| IBIS file usssh2gxxac.ibs created by s2ibis3 verion 1.1
| North Carolina State University, ERL, 2006
| This Model is valid for Commercial Temperature Range 0C<=Tc<=95C
| Valid for DDR3-800/1066/1333/1600/1866 operation
| Part Number   VDD/VDDQ   Package   Architecture
| SCB15H2G160AF   1.5 +0.1/-0.1   96-Ball FBGA   128Meg x 16
| SCB15H2G800AF   1.5 +0.1/-0.1   78-Ball FBGA   256Meg x 8
| TOPR: Operating Temperature
[IBIS Ver]   3.2
[File name]  usssh2gxxac.ibs
[File Rev]   1.2
[Date]   2016-10-18
[Source]   Simulation of a silicon level SPICE model
[Notes]   IBIS Characteristics for I/O Buffer
   IBIS Model Revision History:
Rev 1.1: 2016-03-29
   - IBIS model file initial creation
Rev 1.2: 2016-10-18
   - updata company and other informations;
   - updata OCD rising falling data to support 1866MB frequency;
[disclaimer] The IBIS models are for modeling purpose only and are
   subject to change without any notice. UniIC is not
   responsible for any problems the models may cause.
[Copyright]  Copyright 2016 UniIC Corp. All rights reserved
|   Component SCB15H2G160AF
[Component]   SCB15H2G160AF
[Manufacturer]  UniIC Corp.
| All balls excluding NC, POWER and GND (R[Ohm], L[H], C[F])
[Package]   | 96-Ball FBGA
|Variable   typ   min   max
R_pkg   5.54E-01   4.56E-01   6.22E-01
L_pkg   1.97E-09   1.50E-09   2.61E-09
C_pkg   6.13E-13   3.99E-13   9.02E-13
[Pin] signal_name   model_name   R_pin   L_pin   C_pin
A1   VDDQ   POWER   NA   NA   NA
A2   DQU5   DQ   5.95E-01   1.95E-09   6.80E-13
A3   DQU7   DQ   5.58E-01   1.70E-09   7.16E-13
A7   DQU4   DQ   5.77E-01   1.84E-09   6.35E-13
A8   VDDQ   POWER   NA   NA   NA
A9   VSS   GND   NA   NA   NA
B1   VSSQ   GND   NA   NA   NA
B2   VDD   POWER   NA   NA   NA
B3   VSS   GND   NA   NA   NA
B7   DQSU#   DQ   5.85E-01   2.01E-09   6.55E-13
B8   DQU6   DQ   6.22E-01   2.08E-09   7.44E-13
B9   VSSQ   GND   NA   NA   NA
C1   VDDQ   POWER   NA   NA   NA
C2   DQU3   DQ   5.85E-01   2.21E-09   6.52E-13
C3   DQU1   DQ   5.65E-01   1.96E-09   6.71E-13
C7   DQSU   DQ   5.99E-01   2.17E-09   6.18E-13
C8   DQU2   DQ   5.52E-01   1.73E-09   6.58E-13
C9   VDDQ   POWER   NA   NA   NA
D1   VSSQ   GND   NA   NA   NA
D2   VDDQ   POWER   NA   NA   NA
D3   DMU   DM   5.80E-01   2.01E-09   5.99E-13
D7   DQU0   DQ   5.32E-01   1.62E-09   5.78E-13
D8   VSSQ   GND   NA   NA   NA
D9   VDD   POWER   NA   NA   NA
E1   VSS   GND   NA   NA   NA
E2   VSSQ   GND   NA   NA   NA
E3   DQL0   DQ   5.65E-01   1.98E-09   6.31E-13
E7   DML   DM   5.39E-01   1.73E-09   6.06E-13
E8   VSSQ   GND   NA   NA   NA
E9   VDDQ   POWER   NA   NA   NA
F1   VDDQ   POWER   NA   NA   NA
F2   DQL2   DQ   5.73E-01   2.13E-09   5.09E-13
F3   DQSL   DQ   5.04E-01   2.07E-09   5.92E-13
F7   DQL1   DQ   5.15E-01   1.65E-09   4.09E-13
F8   DQL3   DQ   5.71E-01   1.79E-09   6.63E-13
F9   VSSQ   GND   NA   NA   NA
G1   VSSQ   GND   NA   NA   NA
G2   DQL6   DQ   5.43E-01   1.97E-09   7.24E-13
G3   DQSL#   DQ   5.03E-01   1.93E-09   5.03E-13
G7   VDD   POWER   NA   NA   NA
G8   VSS   GND   NA   NA   NA
G9   VSSQ   GND   NA   NA   NA
H1   VREFDQ   POWER   NA   NA   NA
H2   VDDQ   POWER   NA   NA   NA
H3   DQL4   DQ   4.81E-01   1.70E-09   5.33E-13
H7   DQL7   DQ   5.62E-01   1.79E-09   5.25E-13
H8   DQL5   DQ   5.75E-01   1.70E-09   7.91E-13
H9   VDDQ   POWER   NA   NA   NA
J2   VSS   GND   NA   NA   NA
J3   RAS#   CLKCA_RCV   4.92E-01   1.68E-09   3.99E-13
J7   CK   CLKCA_RCV   4.56E-01   1.60E-09   4.69E-13
J8   VSS   GND   NA   NA   NA
K1   ODT   CLKCA_RCV   5.85E-01   2.12E-09   7.64E-13
K2   VDD   POWER   NA   NA   NA
K3   CAS#   CLKCA_RCV   5.55E-01   1.94E-09   5.21E-13
K7   CK#   CLKCA_RCV   4.58E-01   1.50E-09   4.54E-13
K8   VDD   POWER   NA   NA   NA
K9   CKE   CLKCA_RCV   4.96E-01   1.79E-09   6.88E-13
L2   CS#   CLKCA_RCV   5.74E-01   2.23E-09   7.32E-13
L3   WE#   CLKCA_RCV   5.56E-01   1.92E-09   5.04E-13
L7   A10   CLKCA_RCV   5.69E-01   2.00E-09   4.54E-13
L8   ZQ   NC   5.84E-01   2.14E-09   6.04E-13
M1   VSS   GND   NA   NA   NA
M2   BA0   CLKCA_RCV   5.68E-01   1.89E-09   6.91E-13
M3   BA2   CLKCA_RCV   5.05E-01   1.91E-09   4.65E-13
M8   VREFCA   POWER   NA   NA   NA
M9   VSS   GND   NA   NA   NA
N1   VDD   POWER   NA   NA   NA
N2   A3   CLKCA_RCV   5.78E-01   2.27E-09   6.25E-13
N3   A0   CLKCA_RCV   5.65E-01   2.22E-09   5.42E-13
N7   A12   CLKCA_RCV   4.95E-01   1.93E-09   5.07E-13
N8   BA1   CLKCA_RCV   5.45E-01   2.06E-09   5.77E-13
N9   VDD   POWER   NA   NA   NA
P1   VSS   GND   NA   NA   NA
P2   A5   CLKCA_RCV   5.45E-01   2.08E-09   6.51E-13
P3   A2   CLKCA_RCV   5.82E-01   2.28E-09   5.42E-13
P7   A1   CLKCA_RCV   5.54E-01   2.15E-09   5.86E-13
P8   A4   CLKCA_RCV   5.63E-01   2.07E-09   6.35E-13
P9   VSS   GND   NA   NA   NA
R1   VDD   POWER   NA   NA   NA
R2   A7   CLKCA_RCV   5.84E-01   2.07E-09   6.67E-13
R3   A9   CLKCA_RCV   6.09E-01   2.12E-09   6.50E-13
R7   A11   CLKCA_RCV   5.56E-01   1.91E-09   6.01E-13
R8   A6   CLKCA_RCV   5.89E-01   2.11E-09   8.04E-13
R9   VDD   POWER   NA   NA   NA
T1   VSS   GND   NA   NA   NA
T2   RESET#   CLKCA_RCV   5.46E-01   2.61E-09   9.02E-13
T3   A13   CLKCA_RCV   5.65E-01   2.05E-09   5.96E-13
T8   A8   CLKCA_RCV   6.18E-01   2.40E-09   7.18E-13
T9   VSS   GND   NA   NA   NA
|*****************************  Diff Pin  *************************************
[Diff Pin]  inv_pin  vdiff   tdelay_typ  tdelay_min  tdelay_max
C7   B7   0.30000V   NA   NA   NA
F3   G3   0.30000V   NA   NA   NA
J7   K7   0.30000V   NA   NA   NA
|   Component SCB15H2G800AF
[Component]   SCB15H2G800AF
[Manufacturer]  UniIC Semiconductors Corp.
[Package]   | 78-Ball FBGA
|Variable   typ   min   max
R_pkg   5.57E-01   4.40E-01   6.18E-01
L_pkg   1.87E-09   1.62E-13   2.26E-09
C_pkg   5.84E-13   3.49E-13   8.81E-13
[Pin] signal_name   model_name   R_pin   L_pin   C_pin
A1   VSS   GND   NA   NA   NA
A2   VDD   POWER   NA   NA   NA
A7   NU_TDQS#   NU_TDQS#   6.12E-01   2.01E-09   7.85E-13
A8   VSS   GND   NA   NA   NA
A9   VDD   POWER   NA   NA   NA
B1   VSS   GND   NA   NA   NA
B2   VSSQ   GND   NA   NA   NA
B3   DQ0   DQ   5.90E-01   1.68E-09   6.72E-13
B7   DM_TDQS   DM_TDQS   6.18E-01   1.96E-09   6.83E-13
B8   VSSQ   GND   NA   NA   NA
B9   VDDQ   POWER   NA   NA   NA
C1   VDDQ   POWER   NA   NA   NA
C2   DQ2   DQ   6.08E-01   1.94E-09   7.02E-13
C3   DQS   DQ   5.70E-01   1.97E-09   6.19E-13
C7   DQ1   DQ   6.05E-01   1.83E-09   7.94E-13
C8   DQ3   DQ   5.87E-01   1.73E-09   8.81E-13
C9   VSSQ   GND   NA   NA   NA
D1   VSSQ   GND   NA   NA   NA
D2   DQ6   DQ   5.84E-01   1.77E-09   7.61E-13
D3   DQS#   DQ   5.66E-01   1.84E-09   6.37E-13
D7   VDD   POWER   NA   NA   NA
D8   VSS   GND   NA   NA   NA
D9   VSSQ   GND   NA   NA   NA
E1   VREFDQ   POWER   NA   NA   NA
E2   VDDQ   POWER   NA   NA   NA
E3   DQ4   DQ   6.09E-01   1.83E-09   5.15E-13
E7   DQ7   DQ   5.71E-01   1.73E-09   5.61E-13
E8   DQ5   DQ   6.15E-01   1.76E-09   7.40E-13
E9   VDDQ   POWER   NA   NA   NA
F2   VSS   GND   NA   NA   NA
F3   RAS#   CLKCA_RCV   5.79E-01   1.91E-09   5.82E-13
F7   CK   CLKCA_RCV   5.70E-01   1.97E-09   4.68E-13
F8   VSS   GND   NA   NA   NA
G1   ODT   CLKCA_RCV   5.74E-01   2.03E-09   7.62E-13
G2   VDD   POWER   NA   NA   NA
G3   CAS#   CLKCA_RCV   5.38E-01   1.82E-09   4.48E-13
G7   CK#   CLKCA_RCV   5.67E-01   1.98E-09   5.54E-13
G8   VDD   POWER   NA   NA   NA
G9   CKE   CLKCA_RCV   5.60E-01   1.91E-09   6.95E-13
H2   CS#   CLKCA_RCV   5.95E-01   2.16E-09   4.92E-13
H3   WE#   CLKCA_RCV   5.39E-01   1.88E-09   5.05E-13
H7   A10   CLKCA_RCV   5.32E-01   1.96E-09   4.04E-13
H8   ZQ   NC   5.44E-01   2.02E-09   5.16E-13
J1   VSS   GND   NA   NA   NA
J2   BA0   CLKCA_RCV   5.58E-01   1.62E-09   6.21E-13
J3   BA2   CLKCA_RCV   5.23E-01   1.72E-09   4.22E-13
J8   VREFCA   POWER   NA   NA   NA
J9   VSS   GND   NA   NA   NA
K1   VDD   POWER   NA   NA   NA
K2   A3   CLKCA_RCV   5.35E-01   1.94E-09   5.12E-13
K3   A0   CLKCA_RCV   5.35E-01   1.91E-09   4.86E-13
K7   A12   CLKCA_RCV   5.38E-01   1.82E-09   3.49E-13
K8   BA1   CLKCA_RCV   5.43E-01   1.84E-09   5.86E-13
K9   VDD   POWER   NA   NA   NA
L1   VSS   GND   NA   NA   NA
L2   A5   CLKCA_RCV   5.54E-01   1.99E-09   5.22E-13
L3   A2   CLKCA_RCV   5.49E-01   2.01E-09   3.70E-13
L7   A1   CLKCA_RCV   5.31E-01   1.90E-09   5.05E-13
L8   A4   CLKCA_RCV   5.66E-01   1.77E-09   5.72E-13
L9   VSS   GND   NA   NA   NA
M1   VDD   POWER   NA   NA   NA
M2   A7   CLKCA_RCV   5.32E-01   1.70E-09   6.24E-13
M3   A9   CLKCA_RCV   5.29E-01   1.70E-09   4.68E-13
M7   A11   CLKCA_RCV   5.24E-01   1.84E-09   4.72E-13
M8   A6   CLKCA_RCV   5.15E-01   1.66E-09   6.54E-13
M9   VDD   POWER   NA   NA   NA
N1   VSS   GND   NA   NA   NA
N2   RESET#   CLKCA_RCV   4.40E-01   2.26E-09   7.81E-13
N3   A13   CLKCA_RCV   5.11E-01   1.68E-09   5.74E-13
N7   A14   CLKCA_RCV   5.14E-01   1.67E-09   5.45E-13
N8   A8   CLKCA_RCV   5.39E-01   2.01E-09   5.18E-13
N9   VSS   GND   NA   NA   NA
|*****************************  Diff Pin  *************************************
[Diff Pin]  inv_pin  vdiff   tdelay_typ  tdelay_min  tdelay_max
F7   G7   0.30000V   NA   NA   NA
C3   D3   0.30000V   NA   NA   NA
|B7   A7   0.25000V   NA   NA   NA
|pin B7 and A7 are differential I/O only When TDQS/TDQS#
|is enabled via Mode Register A11=1 in MR1
|If TDQS is disabled, then B7 (DM) is a single
|ended INPUT with ODT and A7 is a NC
|*****************************  Model Selector ********************************
[Model Selector]   DQ
DATA_34_800   RZQ/7 Output Driver (ODT Off & 800Mbps)
DATA_34_1066   RZQ/7 Output Driver (ODT Off & 1066Mbps)
DATA_34_1333   RZQ/7 Output Driver (ODT Off & 1333Mbps)
DATA_34_1600   RZQ/7 Output Driver (ODT Off & 1600Mbps)
DATA_34_1866   RZQ/7 Output Driver (ODT Off & 1866Mbps)
DATA_40_800   RZQ/7 Output Driver (ODT Off & 800Mbps)
DATA_40_1066   RZQ/7 Output Driver (ODT Off & 1066Mbps)
DATA_40_1333   RZQ/7 Output Driver (ODT Off & 1333Mbps)
DATA_40_1600   RZQ/7 Output Driver (ODT Off & 1600Mbps)
DATA_40_1866   RZQ/7 Output Driver (ODT Off & 1866Mbps)
DATA_60_800   RZQ/7 Output Driver (ODT Off & 800Mbps)
DATA_60_1066   RZQ/7 Output Driver (ODT Off & 1066Mbps)
DATA_60_1333   RZQ/7 Output Driver (ODT Off & 1333Mbps)
DATA_60_1600   RZQ/7 Output Driver (ODT Off & 1600Mbps)
DATA_60_1866   RZQ/7 Output Driver (ODT Off & 1866Mbps)
DATA_80_800   RZQ/7 Output Driver (ODT Off & 800Mbps)
DATA_80_1066   RZQ/7 Output Driver (ODT Off & 1066Mbps)
DATA_80_1333   RZQ/7 Output Driver (ODT Off & 1333Mbps)
DATA_80_1600   RZQ/7 Output Driver (ODT Off & 1600Mbps)
DATA_80_1866   RZQ/7 Output Driver (ODT Off & 1866Mbps)
DATA_RCV   Input Model with no ODT
ODT_60   Data Strobe I/O with 60 Ohm ODT (RZQ/4)
ODT_120   Data Strobe I/O with 120 Ohm ODT (RZQ/2)
ODT_40   Data Strobe I/O with 40 Ohm ODT (RZQ/6)
ODT_20   Data Strobe I/O with 20 Ohm ODT (RZQ/12)
ODT_30   Data Strobe I/O with 30 Ohm ODT (RZQ/8)
[Model Selector]   DM
DATA_RCV   Input Model with no ODT
ODT_60   Data Strobe I/O with 60 Ohm ODT (RZQ/4)
ODT_120   Data Strobe I/O with 120 Ohm ODT (RZQ/2)
ODT_40   Data Strobe I/O with 40 Ohm ODT (RZQ/6)
ODT_20   Data Strobe I/O with 20 Ohm ODT (RZQ/12)
ODT_30   Data Strobe I/O with 30 Ohm ODT (RZQ/8)
[Model Selector]   NU_TDQS#
DATA_NC   Non-Functioning Terminator Model
ODT_60   Data Strobe I/O with 60 Ohm ODT (RZQ/4)
ODT_120   Data Strobe I/O with 120 Ohm ODT (RZQ/2)
ODT_40   Data Strobe I/O with 40 Ohm ODT (RZQ/6)
ODT_20   Data Strobe I/O with 20 Ohm ODT (RZQ/12)
ODT_30   Data Strobe I/O with 30 Ohm ODT (RZQ/8)
|When TDQS# is enabled, NU_TDQS# is a output with terminal resistance;
|When TDQS# is disabled, NU_TDQS# is a NC;
[Model Selector]   DM_TDQS
DATA_RCV   Input Model with no ODT
ODT_60   Data Strobe I/O with 60 Ohm ODT (RZQ/4)
ODT_120   Data Strobe I/O with 120 Ohm ODT (RZQ/2)
ODT_40   Data Strobe I/O with 40 Ohm ODT (RZQ/6)
ODT_20   Data Strobe I/O with 20 Ohm ODT (RZQ/12)
ODT_30   Data Strobe I/O with 30 Ohm ODT (RZQ/8)
| Models and submodels in the file (28): DATA_34_800 (I/O), DATA_34_1066 (I/O), DATA_34_1333 (I/O), DATA_34_1600 (I/O), DATA_34_1866 (I/O), DATA_40_800 (I/O), DATA_40_1066 (I/O), DATA_40_1333 (I/O), DATA_40_1600 (I/O), DATA_40_1866 (I/O), DATA_60_800 (I/O), DATA_60_1066 (I/O), DATA_60_1333 (I/O), DATA_60_1600 (I/O), DATA_60_1866 (I/O), DATA_80_800 (I/O), DATA_80_1066 (I/O), DATA_80_1333 (I/O), DATA_80_1600 (I/O), DATA_80_1866 (I/O), DATA_RCV (Input), DATA_NC (Input), ODT_60 (Input), ODT_120 (Input), ODT_40 (Input), ODT_20 (Input), ODT_30 (Input), CLKCA_RCV (Input)
